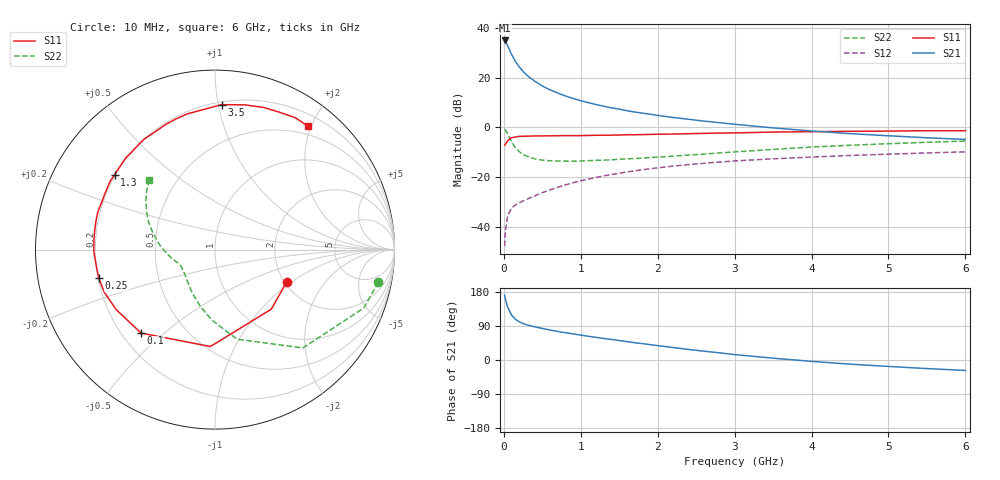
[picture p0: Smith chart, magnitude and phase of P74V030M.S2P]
! SIEMENS Small Signal Semiconductors
! BFP196
! Si NPN RF Bipolar Junction Transistor in SOT143
! VCE = 4 V  IC = 30 mA
! Common Emitter S-Parameters:  May  1996
# GHz  S  MA  R  50
!  f  S11  S21  S12  S22
! GHz  MAG  ANG  MAG  ANG  MAG  ANG  MAG  ANG
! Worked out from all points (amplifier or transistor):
!   36 points, 10 MHz to 6 GHz, reference 50 ohm
!   highest |S21| = 35.0 dB at 10 MHz (marker M1)
!   |S21| within 3 dB of that: start of sweep to 62.41 MHz
!   unconditionally stable (mu >= 1): 572.2 MHz to 3.434 GHz
!   at 250 MHz: K = 0.71, MSG = 26.0 dB, |S12| = -29.5 dB
!   at 1.4 GHz: K = 1.10, MAG = 11.5 dB, |S12| = -18.9 dB
!   at 6 GHz: K = 0.97, MSG = 2.5 dB, |S12| = -9.8 dB
!   lowest NFmin = 1.40 dB at 500 MHz
!   S11 on the Smith chart (normalised r, x): 10 MHz: 2.05, -0.92; 100 MHz: 0.28, -0.42; 250 MHz: 0.20, -0.12; 1.3 GHz: 0.20, +0.32; 3.5 GHz: 0.22, +1.02; 6 GHz: 0.37, +1.94
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0.01  0.4379 -24.3  56.24 170.7  0.0041 78.9  0.9288 -11.3
0.02  0.4567 -46.6  53.47 160.8  0.0081 73.4  0.8898 -21.5
0.05  0.5405 -92.7  43.91 139.2  0.0169 57.7  0.735 -48.2
0.1  0.6211 -131.5  29.6 118.5  0.0239 46.7  0.5146 -76.1
0.15  0.6443 -148.8  21.33 107.6  0.0276 43.9  0.3932 -92.6
0.2  0.6609 -159.0  16.58 100.9  0.0303 44.7  0.3269 -104.4
0.25  0.6669 -166.1  13.36 96.2  0.0334 46.2  0.2858 -113.6
0.3  0.6673 -171.4  11.25 92.8  0.036 48.7  0.2636 -120.3
0.4  0.6753 -179.1  8.555 87.7  0.042 51.5  0.234 -130.9
0.5  0.6765 175.3  6.839 83.3  0.0488 54.6  0.2205 -138.4
0.6  0.6795 170.1  5.723 79.2  0.0557 56.1  0.2142 -143.5
0.7  0.683 165.3  4.924 75.3  0.0627 56.9  0.2116 -147.5
0.8  0.6857 161.8  4.302 72.1  0.07 56.9  0.211 -150.6
1.1  0.6908 150.6  3.15 62.6  0.0919 56.5  0.2151 -157.5
1.3  0.6974 143.4  2.671 56.8  0.1064 55.1  0.2205 -160.9
1.7  0.7145 130.7  2.048 45.6  0.1343 51.1  0.2373 -167.0
2.2  0.736 116.9  1.588 33.0  0.1671 44.6  0.2651 -174.1
3  0.7776 97.3  1.16 14.3  0.212 33.8  0.3221 172.4
3.5  0.8084 87.4  0.981 4.8  0.2344 27.3  0.3623 164.2
4.5  0.8371 71.1  0.752 -10.9  0.2734 15.7  0.4388 150.5
5.5  0.8603 58.7  0.62 -22.6  0.3075 5.0  0.5038 139.0
6  0.8606 53.2  0.576 -27.6  0.3239 -0.8  0.5332 133.3
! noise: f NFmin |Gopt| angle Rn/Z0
0.5  1.4  0.4  -173  0.08
0.9  1.6  0.5  -166  0.08
1.5  2.4  0.61  -150  0.14
2  2.9  0.71  -129  0.2
